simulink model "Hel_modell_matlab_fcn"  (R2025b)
settings: Solver=VariableStepAuto  StartTime=0.0  StopTime=10.0  RelTol=1e-3
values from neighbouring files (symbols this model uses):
  AFs = 14.6    [Lektion_2.m]
  eta_vol = 0.8    [Lektion_2.m]
  Je = 0.1    [Lektion_2.m]
  Ki = 0.1    [Lektion_2.m]
  Kp = 0    [Lektion_2.m]
  m_dot_a_end = 18*1e-3    (= 0.018)    [Lektion_2.m]
  m_dot_a_start = 12*1e-3    (= 0.012)    [Lektion_2.m]
  m_dot_fi_start = m_dot_a_start/AFs    (= 0.000821917808219)    [Lektion_2.m]
  m_th_1 = 12/1000    (= 0.012)    [Lektion_2.m]
  n_cyl = 4    [Lektion_2.m]
  N_init = 3000/60    (= 50)    [Lektion_2.m]
  n_r = 2    [Lektion_2.m]
  R = 280    [Lektion_2.m]
  T_i = 320    [Lektion_2.m]
  tau_d = 0.2    [Lektion_2.m]
  tau_mix = 0.14    [Lektion_2.m]
  tau_sensor = 0.05    [Lektion_2.m]
  tau_th = 1/0.1    (= 10)    [Lektion_2.m]
  V_d = 0.55/1e3    (= 0.00055)    [Lektion_2.m]
  V_i = 2/1e3    (= 0.002)    [Lektion_2.m]
undefined symbols (not defined in the file or in its folder): p_im

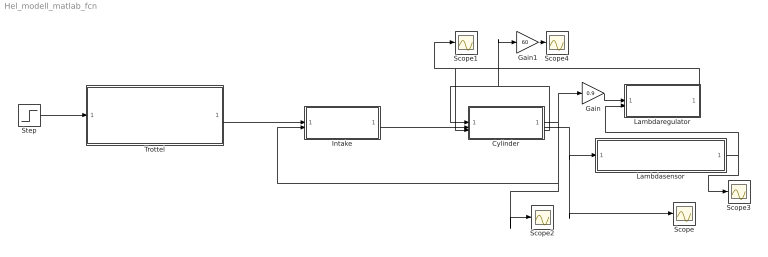
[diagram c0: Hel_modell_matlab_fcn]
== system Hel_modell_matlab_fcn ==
  Cylinder : Subsystem
  Gain : Gain  Gain=0.9
  Gain1 : Gain  Gain=60
  Intake : Subsystem
  Lambdaregulator : Subsystem
  Lambdasensor : Subsystem
  Scope{,1..4} (5 alike) : Scope
  Step : Step  Time=5  Before=m_dot_a_start  After=m_dot_a_end  SampleTime=0
  Trottel : Subsystem
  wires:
  Cylinder/1(m_ac [kg/s]) -> Intake/2(m_ac [kg/s]), Scope2/1, Gain/1
  Step/1 -> Trottel/1(m_at,raf [kg/s])
  Trottel/1(m_at [kg/s]) -> Intake/1(m_at [kg/s])
  Intake/1(p_im [Pa]) -> Cylinder/2(p_im [Pa])
  Cylinder/3(N_e [rps]) -> Gain1/1, Cylinder/1(N [rps])
  Lambdaregulator/1(m_fi [kg/s]) -> Cylinder/3(m_fi [kg/s]), Scope1/1
  Cylinder/2(lambda_c [-]) -> Scope/1, Lambdasensor/1(lambda_c [-])
  Lambdasensor/1(lambda_d [-]) -> Lambdaregulator/2(lambda_d [-]), Scope3/1
  Gain/1 -> Lambdaregulator/1(m_ac_mod)
  Gain1/1 -> Scope4/1

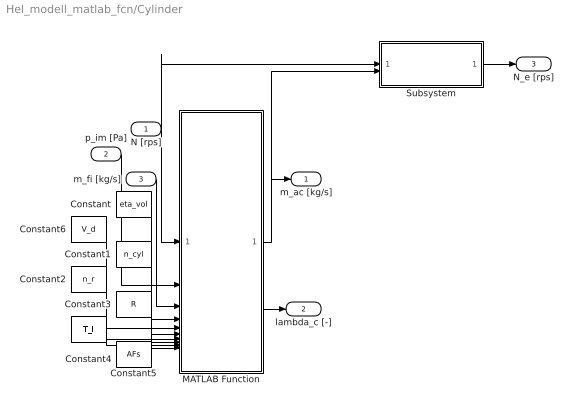
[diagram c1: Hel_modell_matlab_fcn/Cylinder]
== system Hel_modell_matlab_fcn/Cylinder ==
  N [rps] : Inport
  p_im [Pa] : Inport  Port=2
  m_fi [kg/s] : Inport  Port=3
  Constant : Constant  Value=eta_vol
  Constant1 : Constant  Value=n_cyl
  Constant2 : Constant  Value=n_r
  Constant3 : Constant  Value=R
  Constant4 : Constant  Value=T_i
  Constant5 : Constant  Value=AFs
  Constant6 : Constant  Value=V_d
  MATLAB Function : MATLAB Function  TreatAsAtomicUnit=on
  Subsystem : Subsystem
  m_ac [kg/s] : Outport
  lambda_c [-] : Outport  Port=2
  N_e [rps] : Outport  Port=3
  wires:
  N [rps]/1 -> Subsystem/1(N [rps]), MATLAB Function/1(N)
  Subsystem/1(N_e [rps]) -> N_e [rps]/1
  MATLAB Function/2(lambda) -> lambda_c [-]/1
  m_fi [kg/s]/1 -> MATLAB Function/3(m_fi)
  p_im [Pa]/1 -> MATLAB Function/2(p_im)
  Constant3/1 -> MATLAB Function/8(R)
  Constant4/1 -> MATLAB Function/9(T)
  Constant2/1 -> MATLAB Function/7(n_r)
  Constant5/1 -> MATLAB Function/10(AFs)
  Constant1/1 -> MATLAB Function/6(n_cyl)
  Constant6/1 -> MATLAB Function/5(V_d)
  Constant/1 -> MATLAB Function/4(eta_vol)
  MATLAB Function/1(m_ac) -> Subsystem/2(m_ac [kg/s]), m_ac [kg/s]/1

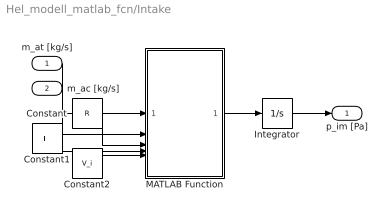
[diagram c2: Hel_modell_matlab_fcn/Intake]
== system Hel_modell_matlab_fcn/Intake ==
  m_at [kg/s] : Inport
  m_ac [kg/s] : Inport  Port=2
  Constant : Constant  Value=R
  Constant1 : Constant  Value=T_i
  Constant2 : Constant  Value=V_i
  Integrator : Integrator  InitialCondition=p_im
  MATLAB Function : MATLAB Function  TreatAsAtomicUnit=on
  p_im [Pa] : Outport
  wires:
  Integrator/1 -> p_im [Pa]/1
  MATLAB Function/1(y) -> Integrator/1
  m_ac [kg/s]/1 -> MATLAB Function/2(m_ac)
  m_at [kg/s]/1 -> MATLAB Function/1(m_at)
  Constant/1 -> MATLAB Function/3(R)
  Constant1/1 -> MATLAB Function/4(T)
  Constant2/1 -> MATLAB Function/5(V)

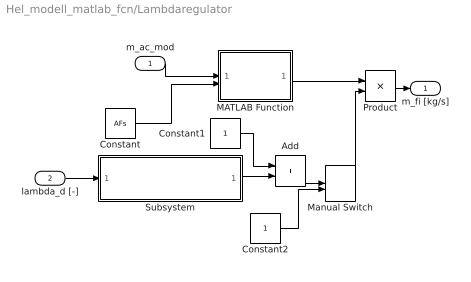
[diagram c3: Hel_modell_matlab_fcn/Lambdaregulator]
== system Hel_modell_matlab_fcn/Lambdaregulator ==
  m_ac_mod : Inport
  lambda_d [-] : Inport  Port=2
  Add : Sum
  Constant : Constant  Value=AFs
  Constant1 : Constant
  Constant2 : Constant
  MATLAB Function : MATLAB Function  TreatAsAtomicUnit=on
  Manual Switch : ManualSwitch
  Product : Product
  Subsystem : Subsystem
  m_fi [kg/s] : Outport
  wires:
  m_ac_mod/1 -> MATLAB Function/1(m_ac)
  Constant/1 -> MATLAB Function/2(AFs)
  Constant1/1 -> Add/1
  MATLAB Function/1(m_fi) -> Product/1
  Product/1 -> m_fi [kg/s]/1
  Subsystem/1("Lambda_controlled ") -> Add/2
  lambda_d [-]/1 -> Subsystem/1(lambda_d)
  Add/1 -> Manual Switch/1
  Manual Switch/1 -> Product/2
  Constant2/1 -> Manual Switch/2

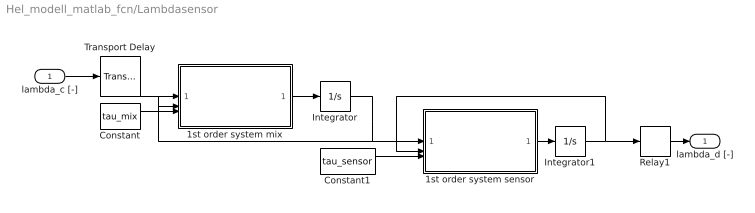
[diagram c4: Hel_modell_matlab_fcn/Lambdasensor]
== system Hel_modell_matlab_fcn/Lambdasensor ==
  lambda_c [-] : Inport
  1st order system mix : MATLAB Function  TreatAsAtomicUnit=on
  1st order system sensor : MATLAB Function  TreatAsAtomicUnit=on
  Constant : Constant  Value=tau_mix
  Constant1 : Constant  Value=tau_sensor
  Integrator : Integrator  InitialCondition=0.8
  Integrator1 : Integrator  InitialCondition=0.8
  Relay1 : Relay  OnSwitchValue=1+eps  OffSwitchValue=1-eps
  Transport Delay : TransportDelay  DelayTime=tau_d  InitialOutput=0.8
  lambda_d [-] : Outport
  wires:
  Integrator1/1 -> 1st order system sensor/2(actual), Relay1/1
  Relay1/1 -> lambda_d [-]/1
  1st order system sensor/1(alpha) -> Integrator1/1
  lambda_c [-]/1 -> Transport Delay/1
  1st order system mix/1(alpha) -> Integrator/1
  Constant1/1 -> 1st order system sensor/3(tau)
  Transport Delay/1 -> 1st order system mix/1(ref)
  Constant/1 -> 1st order system mix/3(tau)
  Integrator/1 -> 1st order system sensor/1(ref), 1st order system mix/2(actual)

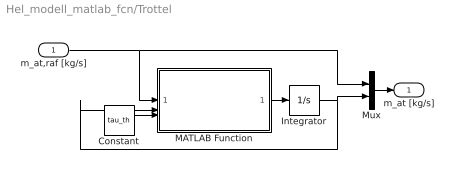
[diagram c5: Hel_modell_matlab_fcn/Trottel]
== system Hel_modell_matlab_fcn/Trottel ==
  m_at,raf [kg/s] : Inport
  Constant : Constant  Value=tau_th
  Integrator : Integrator  InitialCondition=m_th_1
  MATLAB Function : MATLAB Function  TreatAsAtomicUnit=on
  Mux : Mux  Inputs=2
  m_at [kg/s] : Outport
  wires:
  Integrator/1 -> MATLAB Function/2(actual), Mux/2
  Mux/1 -> m_at [kg/s]/1
  m_at,raf [kg/s]/1 -> MATLAB Function/1(ref), Mux/1
  MATLAB Function/1(alpha) -> Integrator/1
  Constant/1 -> MATLAB Function/3(tau)

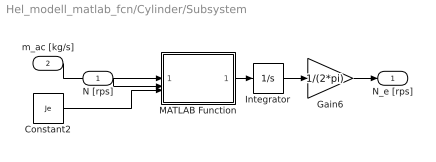
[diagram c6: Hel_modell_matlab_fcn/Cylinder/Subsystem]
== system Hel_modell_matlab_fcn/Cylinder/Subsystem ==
  N [rps] : Inport
  m_ac [kg/s] : Inport  Port=2
  Constant2 : Constant  Value=Je
  Gain6 : Gain  Gain=1/(2*pi)
  Integrator : Integrator  InitialCondition=N_init*2*pi
  MATLAB Function : MATLAB Function  TreatAsAtomicUnit=on
  N_e [rps] : Outport
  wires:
  Integrator/1 -> Gain6/1
  Gain6/1 -> N_e [rps]/1
  Constant2/1 -> MATLAB Function/3(Je)
  N [rps]/1 -> MATLAB Function/2(N)
  m_ac [kg/s]/1 -> MATLAB Function/1(m_ac_dot)
  MATLAB Function/1(w_m_dot) -> Integrator/1

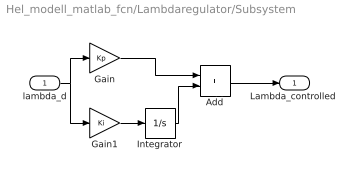
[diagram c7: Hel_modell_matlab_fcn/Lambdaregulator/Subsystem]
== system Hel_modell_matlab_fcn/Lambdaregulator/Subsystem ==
  lambda_d : Inport
  Add : Sum
  Gain : Gain  Gain=Kp
  Gain1 : Gain  Gain=Ki
  Integrator : Integrator  InitialCondition=m_dot_fi_start
  "Lambda_controlled " : Outport
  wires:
  Add/1 -> "Lambda_controlled "/1
  Gain1/1 -> Integrator/1
  Integrator/1 -> Add/2
  lambda_d/1 -> Gain/1, Gain1/1
  Gain/1 -> Add/1

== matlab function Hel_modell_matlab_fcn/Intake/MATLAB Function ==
function y = fcn(m_at,m_ac,R,T,V)

y = u;

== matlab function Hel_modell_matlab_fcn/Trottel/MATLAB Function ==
function alpha = fcn(ref, actual, tau)
error = ref - actual;

alpha =  error*tau;

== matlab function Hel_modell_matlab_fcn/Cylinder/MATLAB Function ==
function [m_ac, lambda]= fcn(N, p_im, m_fi,eta_vol,V_d,n_cyl,n_r,R,T,AFs)

m_ac = eta_vol*N*p_im*V_d*n_cyl/(n_r*R*T);

lambda = m_ac/m_fi * 1/AFs;

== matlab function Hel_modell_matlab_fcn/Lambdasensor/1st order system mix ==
function alpha = fcn(ref, actual, tau)
error = ref - actual;

alpha =  error*tau;

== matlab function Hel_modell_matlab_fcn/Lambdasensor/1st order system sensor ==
function alpha = fcn(ref, actual, tau)
error = ref - actual;

alpha =  error*tau;

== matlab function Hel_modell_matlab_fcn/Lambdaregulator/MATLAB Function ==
function m_fi = fcn(m_ac, AFs)

m_fi = m_ac/AFs;

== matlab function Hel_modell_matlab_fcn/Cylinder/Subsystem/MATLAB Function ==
function w_m_dot = fcn(m_ac_dot, N, Je)

m_ac = m_ac_dot/N;

Me = 3.3402*10^10 * m_ac^3 - 1.1409*10^8 * m_ac^2 + 2.4357*10^5 * m_ac - 54.567;

Mb = 0.42*N + 0.0036*N^2;

w_m_dot = (Me-Mb)/Je;
